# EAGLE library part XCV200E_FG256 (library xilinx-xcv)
xcv200e_fg256 edit this description Auto generated by make-symbol-device-package-bsdl.ulp Rev. 26 Source: xcv200e_fg256.bsd
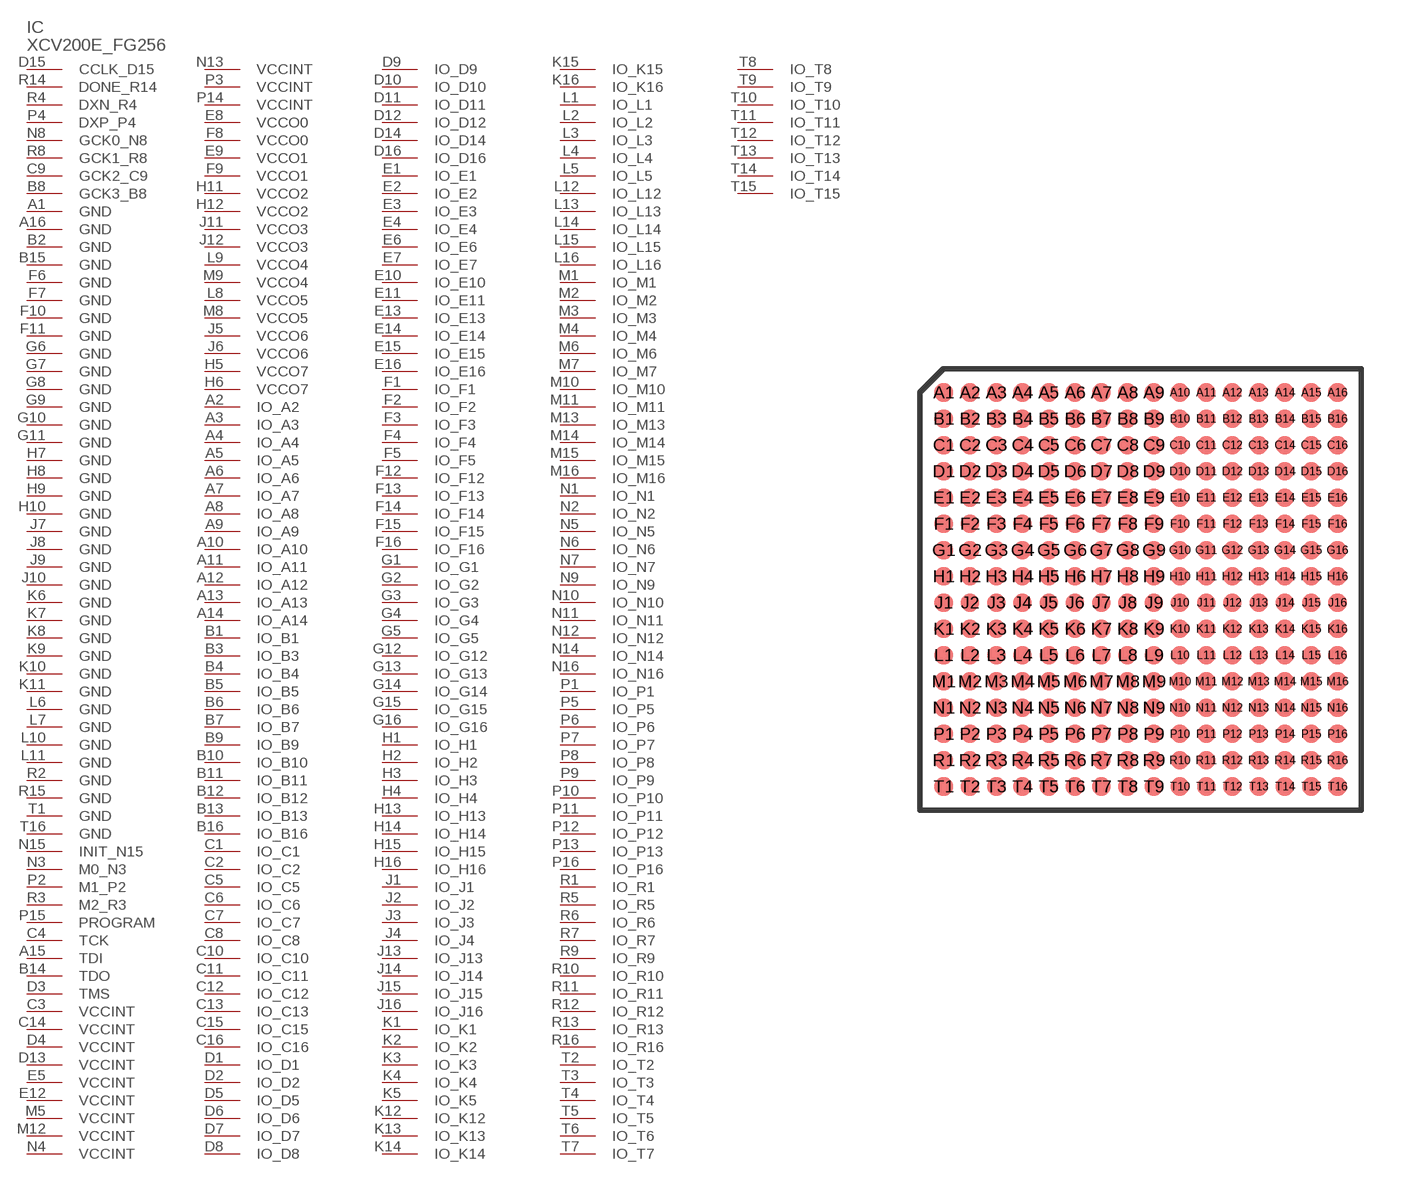
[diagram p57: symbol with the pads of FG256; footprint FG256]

Designator prefix IC

## XCV200E_FG256 (OC_FARNELL: unknown; OC_NEWARK: unknown)  [FG256]
A1  GND  pwr
A2  IO_A2
A3  IO_A3
A4  IO_A4
A5  IO_A5
A6  IO_A6
A7  IO_A7
A8  IO_A8
A9  IO_A9
A10  IO_A10
A11  IO_A11
A12  IO_A12
A13  IO_A13
A14  IO_A14
A15  TDI  in
A16  GND  pwr
B1  IO_B1
B2  GND  pwr
B3  IO_B3
B4  IO_B4
B5  IO_B5
B6  IO_B6
B7  IO_B7
B8  GCK3_B8  in
B9  IO_B9
B10  IO_B10
B11  IO_B11
B12  IO_B12
B13  IO_B13
B14  TDO  out
B15  GND  pwr
B16  IO_B16
C1  IO_C1
C2  IO_C2
C3  VCCINT  pwr
C4  TCK  in
C5  IO_C5
C6  IO_C6
C7  IO_C7
C8  IO_C8
C9  GCK2_C9  in
C10  IO_C10
C11  IO_C11
C12  IO_C12
C13  IO_C13
C14  VCCINT  pwr
C15  IO_C15
C16  IO_C16
D1  IO_D1
D2  IO_D2
D3  TMS  in
D4  VCCINT  pwr
D5  IO_D5
D6  IO_D6
D7  IO_D7
D8  IO_D8
D9  IO_D9
D10  IO_D10
D11  IO_D11
D12  IO_D12
D13  VCCINT  pwr
D14  IO_D14
D15  CCLK_D15
D16  IO_D16
E1  IO_E1
E2  IO_E2
E3  IO_E3
E4  IO_E4
E5  VCCINT  pwr
E6  IO_E6
E7  IO_E7
E8  VCCO0  pwr
E9  VCCO1  pwr
E10  IO_E10
E11  IO_E11
E12  VCCINT  pwr
E13  IO_E13
E14  IO_E14
E15  IO_E15
E16  IO_E16
F1  IO_F1
F2  IO_F2
F3  IO_F3
F4  IO_F4
F5  IO_F5
F6  GND  pwr
F7  GND  pwr
F8  VCCO0  pwr
F9  VCCO1  pwr
F10  GND  pwr
F11  GND  pwr
F12  IO_F12
F13  IO_F13
F14  IO_F14
F15  IO_F15
F16  IO_F16
G1  IO_G1
G2  IO_G2
G3  IO_G3
G4  IO_G4
G5  IO_G5
G6  GND  pwr
G7  GND  pwr
G8  GND  pwr
G9  GND  pwr
G10  GND  pwr
G11  GND  pwr
G12  IO_G12
G13  IO_G13
G14  IO_G14
G15  IO_G15
G16  IO_G16
H1  IO_H1
H2  IO_H2
H3  IO_H3
H4  IO_H4
H5  VCCO7  pwr
H6  VCCO7  pwr
H7  GND  pwr
H8  GND  pwr
H9  GND  pwr
H10  GND  pwr
H11  VCCO2  pwr
H12  VCCO2  pwr
H13  IO_H13
H14  IO_H14
H15  IO_H15
H16  IO_H16
J1  IO_J1
J2  IO_J2
J3  IO_J3
J4  IO_J4
J5  VCCO6  pwr
J6  VCCO6  pwr
J7  GND  pwr
J8  GND  pwr
J9  GND  pwr
J10  GND  pwr
J11  VCCO3  pwr
J12  VCCO3  pwr
J13  IO_J13
J14  IO_J14
J15  IO_J15
J16  IO_J16
K1  IO_K1
K2  IO_K2
K3  IO_K3
K4  IO_K4
K5  IO_K5
K6  GND  pwr
K7  GND  pwr
K8  GND  pwr
K9  GND  pwr
K10  GND  pwr
K11  GND  pwr
K12  IO_K12
K13  IO_K13
K14  IO_K14
K15  IO_K15
K16  IO_K16
L1  IO_L1
L2  IO_L2
L3  IO_L3
L4  IO_L4
L5  IO_L5
L6  GND  pwr
L7  GND  pwr
L8  VCCO5  pwr
L9  VCCO4  pwr
L10  GND  pwr
L11  GND  pwr
L12  IO_L12
L13  IO_L13
L14  IO_L14
L15  IO_L15
L16  IO_L16
M1  IO_M1
M2  IO_M2
M3  IO_M3
M4  IO_M4
M5  VCCINT  pwr
M6  IO_M6
M7  IO_M7
M8  VCCO5  pwr
M9  VCCO4  pwr
M10  IO_M10
M11  IO_M11
M12  VCCINT  pwr
M13  IO_M13
M14  IO_M14
M15  IO_M15
M16  IO_M16
N1  IO_N1
N2  IO_N2
N3  M0_N3  in
N4  VCCINT  pwr
N5  IO_N5
N6  IO_N6
N7  IO_N7
N8  GCK0_N8  in
N9  IO_N9
N10  IO_N10
N11  IO_N11
N12  IO_N12
N13  VCCINT  pwr
N14  IO_N14
N15  INIT_N15
N16  IO_N16
P1  IO_P1
P2  M1_P2  in
P3  VCCINT  pwr
P4  DXP_P4  pas
P5  IO_P5
P6  IO_P6
P7  IO_P7
P8  IO_P8
P9  IO_P9
P10  IO_P10
P11  IO_P11
P12  IO_P12
P13  IO_P13
P14  VCCINT  pwr
P15  PROGRAM  in
P16  IO_P16
R1  IO_R1
R2  GND  pwr
R3  M2_R3  in
R4  DXN_R4  pas
R5  IO_R5
R6  IO_R6
R7  IO_R7
R8  GCK1_R8  in
R9  IO_R9
R10  IO_R10
R11  IO_R11
R12  IO_R12
R13  IO_R13
R14  DONE_R14
R15  GND  pwr
R16  IO_R16
T1  GND  pwr
T2  IO_T2
T3  IO_T3
T4  IO_T4
T5  IO_T5
T6  IO_T6
T7  IO_T7
T8  IO_T8
T9  IO_T9
T10  IO_T10
T11  IO_T11
T12  IO_T12
T13  IO_T13
T14  IO_T14
T15  IO_T15
T16  GND  pwr

## Footprint FG256 (pad centres in mm)
Fine Pitch BGA (FG256) Auto generated by make-symbol-device-package-bsdl.ulp Rev. 26 Source: xcv100_fg256.bsd; fg256.pdf
smd 0.7 x 0.7: A1 -7.5,7.5; A2 -6.5,7.5; A3 -5.5,7.5; A4 -4.5,7.5; A5 -3.5,7.5; A6 -2.5,7.5; A7 -1.5,7.5; A8 -0.5,7.5; A9 0.5,7.5; A10 1.5,7.5; A11 2.5,7.5; A12 3.5,7.5; A13 4.5,7.5; A14 5.5,7.5; A15 6.5,7.5; A16 7.5,7.5; B1 -7.5,6.5; B2 -6.5,6.5; B3 -5.5,6.5; B4 -4.5,6.5; B5 -3.5,6.5; B6 -2.5,6.5; B7 -1.5,6.5; B8 -0.5,6.5; B9 0.5,6.5; B10 1.5,6.5; B11 2.5,6.5; B12 3.5,6.5; B13 4.5,6.5; B14 5.5,6.5; B15 6.5,6.5; B16 7.5,6.5; C1 -7.5,5.5; C2 -6.5,5.5; C3 -5.5,5.5; C4 -4.5,5.5; C5 -3.5,5.5; C6 -2.5,5.5; C7 -1.5,5.5; C8 -0.5,5.5; C9 0.5,5.5; C10 1.5,5.5; C11 2.5,5.5; C12 3.5,5.5; C13 4.5,5.5; C14 5.5,5.5; C15 6.5,5.5; C16 7.5,5.5; D1 -7.5,4.5; D2 -6.5,4.5; D3 -5.5,4.5; D4 -4.5,4.5; D5 -3.5,4.5; D6 -2.5,4.5; D7 -1.5,4.5; D8 -0.5,4.5; D9 0.5,4.5; D10 1.5,4.5; D11 2.5,4.5; D12 3.5,4.5; D13 4.5,4.5; D14 5.5,4.5; D15 6.5,4.5; D16 7.5,4.5; E1 -7.5,3.5; E2 -6.5,3.5; E3 -5.5,3.5; E4 -4.5,3.5; E5 -3.5,3.5; E6 -2.5,3.5; E7 -1.5,3.5; E8 -0.5,3.5; E9 0.5,3.5; E10 1.5,3.5; E11 2.5,3.5; E12 3.5,3.5; E13 4.5,3.5; E14 5.5,3.5; E15 6.5,3.5; E16 7.5,3.5; F1 -7.5,2.5; F2 -6.5,2.5; F3 -5.5,2.5; F4 -4.5,2.5; F5 -3.5,2.5; F6 -2.5,2.5; F7 -1.5,2.5; F8 -0.5,2.5; F9 0.5,2.5; F10 1.5,2.5; F11 2.5,2.5; F12 3.5,2.5; F13 4.5,2.5; F14 5.5,2.5; F15 6.5,2.5; F16 7.5,2.5; G1 -7.5,1.5; G2 -6.5,1.5; G3 -5.5,1.5; G4 -4.5,1.5; G5 -3.5,1.5; G6 -2.5,1.5; G7 -1.5,1.5; G8 -0.5,1.5; G9 0.5,1.5; G10 1.5,1.5; G11 2.5,1.5; G12 3.5,1.5; G13 4.5,1.5; G14 5.5,1.5; G15 6.5,1.5; G16 7.5,1.5; H1 -7.5,0.5; H2 -6.5,0.5; H3 -5.5,0.5; H4 -4.5,0.5; H5 -3.5,0.5; H6 -2.5,0.5; H7 -1.5,0.5; H8 -0.5,0.5; H9 0.5,0.5; H10 1.5,0.5; H11 2.5,0.5; H12 3.5,0.5; H13 4.5,0.5; H14 5.5,0.5; H15 6.5,0.5; H16 7.5,0.5; J1 -7.5,-0.5; J2 -6.5,-0.5; J3 -5.5,-0.5; J4 -4.5,-0.5; J5 -3.5,-0.5; J6 -2.5,-0.5; J7 -1.5,-0.5; J8 -0.5,-0.5; J9 0.5,-0.5; J10 1.5,-0.5; J11 2.5,-0.5; J12 3.5,-0.5; J13 4.5,-0.5; J14 5.5,-0.5; J15 6.5,-0.5; J16 7.5,-0.5; K1 -7.5,-1.5; K2 -6.5,-1.5; K3 -5.5,-1.5; K4 -4.5,-1.5; K5 -3.5,-1.5; K6 -2.5,-1.5; K7 -1.5,-1.5; K8 -0.5,-1.5; K9 0.5,-1.5; K10 1.5,-1.5; K11 2.5,-1.5; K12 3.5,-1.5; K13 4.5,-1.5; K14 5.5,-1.5; K15 6.5,-1.5; K16 7.5,-1.5; L1 -7.5,-2.5; L2 -6.5,-2.5; L3 -5.5,-2.5; L4 -4.5,-2.5; L5 -3.5,-2.5; L6 -2.5,-2.5; L7 -1.5,-2.5; L8 -0.5,-2.5; L9 0.5,-2.5; L10 1.5,-2.5; L11 2.5,-2.5; L12 3.5,-2.5; L13 4.5,-2.5; L14 5.5,-2.5; L15 6.5,-2.5; L16 7.5,-2.5; M1 -7.5,-3.5; M2 -6.5,-3.5; M3 -5.5,-3.5; M4 -4.5,-3.5; M5 -3.5,-3.5; M6 -2.5,-3.5; M7 -1.5,-3.5; M8 -0.5,-3.5; M9 0.5,-3.5; M10 1.5,-3.5; M11 2.5,-3.5; M12 3.5,-3.5; M13 4.5,-3.5; M14 5.5,-3.5; M15 6.5,-3.5; M16 7.5,-3.5; N1 -7.5,-4.5; N2 -6.5,-4.5; N3 -5.5,-4.5; N4 -4.5,-4.5; N5 -3.5,-4.5; N6 -2.5,-4.5; N7 -1.5,-4.5; N8 -0.5,-4.5; N9 0.5,-4.5; N10 1.5,-4.5; N11 2.5,-4.5; N12 3.5,-4.5; N13 4.5,-4.5; N14 5.5,-4.5; N15 6.5,-4.5; N16 7.5,-4.5; P1 -7.5,-5.5; P2 -6.5,-5.5; P3 -5.5,-5.5; P4 -4.5,-5.5; P5 -3.5,-5.5; P6 -2.5,-5.5; P7 -1.5,-5.5; P8 -0.5,-5.5; P9 0.5,-5.5; P10 1.5,-5.5; P11 2.5,-5.5; P12 3.5,-5.5; P13 4.5,-5.5; P14 5.5,-5.5; P15 6.5,-5.5; P16 7.5,-5.5; R1 -7.5,-6.5; R2 -6.5,-6.5; R3 -5.5,-6.5; R4 -4.5,-6.5; R5 -3.5,-6.5; R6 -2.5,-6.5; R7 -1.5,-6.5; R8 -0.5,-6.5; R9 0.5,-6.5; R10 1.5,-6.5; R11 2.5,-6.5; R12 3.5,-6.5; R13 4.5,-6.5; R14 5.5,-6.5; R15 6.5,-6.5; R16 7.5,-6.5; T1 -7.5,-7.5; T2 -6.5,-7.5; T3 -5.5,-7.5; T4 -4.5,-7.5; T5 -3.5,-7.5; T6 -2.5,-7.5; T7 -1.5,-7.5; T8 -0.5,-7.5; T9 0.5,-7.5; T10 1.5,-7.5; T11 2.5,-7.5; T12 3.5,-7.5; T13 4.5,-7.5; T14 5.5,-7.5; T15 6.5,-7.5; T16 7.5,-7.5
